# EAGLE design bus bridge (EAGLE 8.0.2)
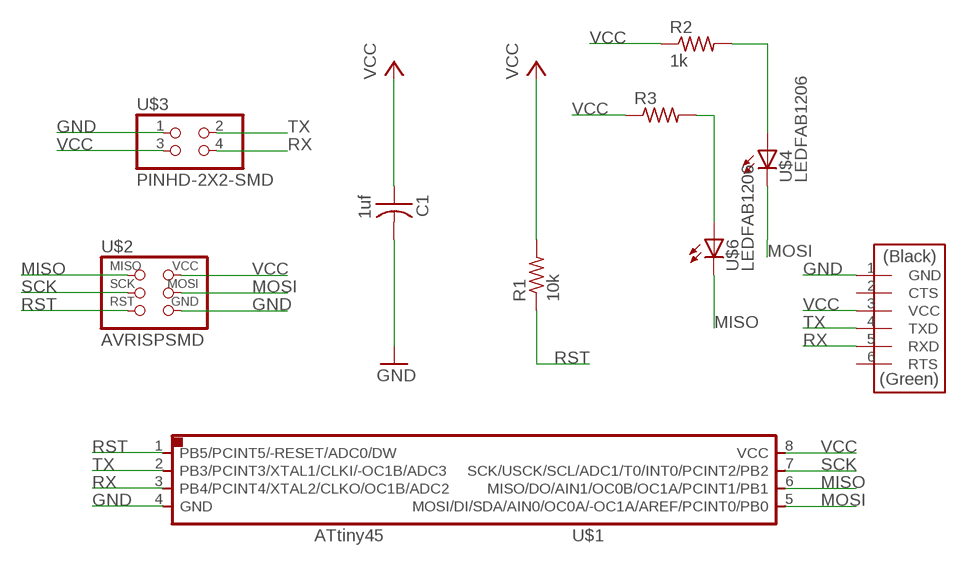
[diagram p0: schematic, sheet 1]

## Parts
C1  1uf  CAP-US1206FAB  [C1206FAB]
R1  10k  RES-US1206FAB  [R1206FAB]
R2  1k  RES-US1206FAB  [R1206FAB]
R3  RES-US1206FAB  [R1206FAB]
U$1  ATTINY45SI  [SOIC8]
U$2  AVRISPSMD  [2X03SMD]
U$3  PINHD-2X2-SMD  [2X02SMD]
U$4  LEDFAB1206  [LED1206FAB]
U$5  FTDI-SMD-HEADER  [1X06SMD]
U$6  LEDFAB1206  [LED1206FAB]

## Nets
GND: C1.2 U$1.4(GND) U$2.6(GND) U$3.1 U$5.1(GND)
MISO: U$1.6(MISO/DO/AIN1/OC0B/OC1A/PCINT1/PB1) U$2.1(MISO) U$6.2(C)
MOSI: U$1.5(MOSI/DI/SDA/AIN0/OC0A/-OC1A/AREF/PCINT0/PB0) U$2.4(MOSI) U$4.2(C)
N$2: R2.2 U$4.1(A)
N$3: R3.2 U$6.1(A)
RST: R1.1 U$1.1(PB5/PCINT5/-RESET/ADC0/DW) U$2.5(RST)
RX: U$1.3(PB4/PCINT4/XTAL2/CLKO/OC1B/ADC2) U$3.4 U$5.5(RXD)
SCK: U$1.7(SCK/USCK/SCL/ADC1/T0/INT0/PCINT2/PB2) U$2.3(SCK)
TX: U$1.2(PB3/PCINT3/XTAL1/CLKI/-OC1B/ADC3) U$3.2 U$5.4(TXD)
VCC: C1.1 R1.2 R2.1 R3.1 U$1.8(VCC) U$2.2(VCC) U$3.3 U$5.3(VCC)
Unconnected: U$5.2(CTS) U$5.6(RTS)

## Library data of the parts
C1 = fab:CAP-US
R1-R3 = fab:RES-US: Resistor (US Symbol)
U$1 = fab:ATTINY45
U$2 = fab:AVRISP
U$3 = fab:PINHD-2X2-SMD
U$4 U$6 = fab:LED: LED
U$5 = fab:FTDI-SMD-HEADER

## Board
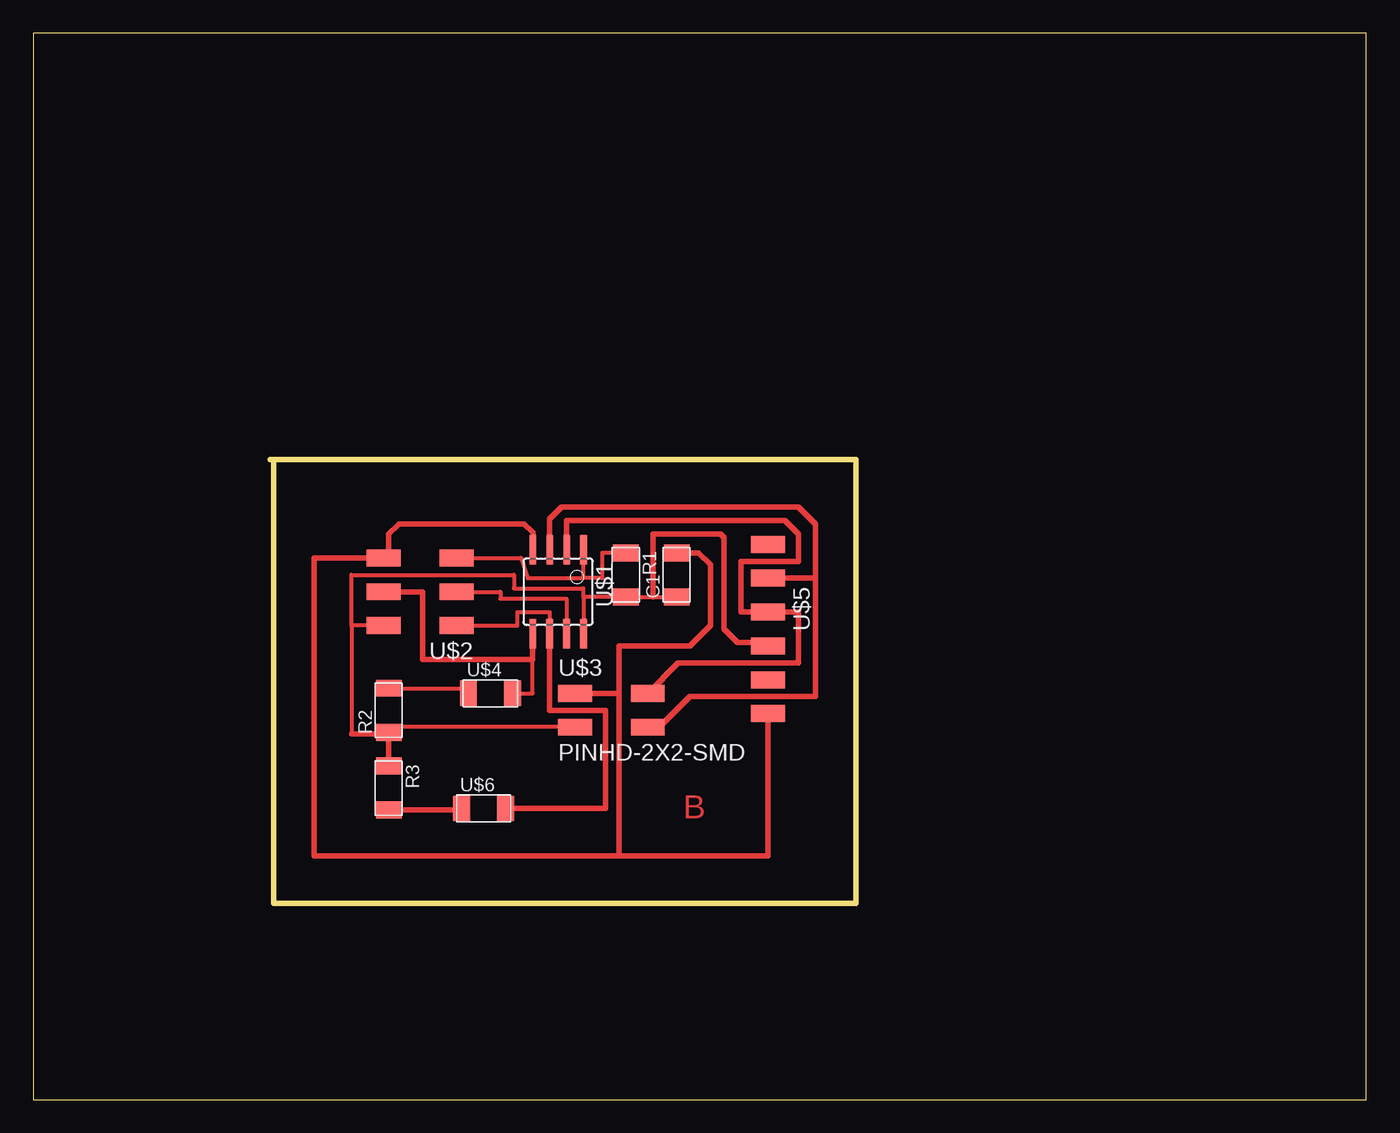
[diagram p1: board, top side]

Size 100 x 80 mm. Coordinates in mm from the lower left corner, seen from the top.
Outline: 17.78,48.01 61.72,48.01 61.72,14.73 18.03,14.73 18.03,47.75
Outline: 0,0 100,0 100,80 0,80 0,0
Copper layers (1*16): Top 0.035mm / dielectric 1.5mm / Bottom 0.035mm
Design rules "default": minimum track width 10mil, minimum drill 24mil, track to track 8mil, track to pad 8mil, pad to pad 8mil, via to via 8mil, smd to smd 8mil, copper to edge 40mil, drill to drill 8mil, minimum pad ring 10mil, minimum via ring 8mil, stop-mask expansion 4mil, vias tented up to drill 0mil, thermal gap 10mil

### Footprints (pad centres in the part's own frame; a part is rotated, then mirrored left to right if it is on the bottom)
C1206FAB = smd 1.27 x 1.905: 1 -1.651,0; 2 1.651,0
R1206FAB = smd 1.27 x 1.905: 1 -1.651,0; 2 1.651,0
SOIC8 = smd 0.5 x 2.2: 1 -1.905,-3.154; 2 -0.645,-3.154; 3 0.625,-3.154; 4 1.895,-3.154; 5 1.905,3.154; 6 0.635,3.154; 7 -0.635,3.154; 8 -1.905,3.154
2X03SMD = smd 2.54 x 1.27: 1 -2.54,2.54; 2 2.92,2.54; 3 -2.54,0; 4 2.92,0; 5 -2.54,-2.54; 6 2.92,-2.54
2X02SMD = smd 2.54 x 1.27: 1 -2.54,1.27; 2 2.92,1.27; 3 -2.54,-1.27; 4 2.92,-1.27
LED1206FAB = smd 1.27 x 1.905: 1 -1.651,0; 2 1.651,0
1X06SMD = smd 2.54 x 1.27: 1 0,6.35; 2 0,3.81; 3 0,1.27; 4 0,-1.27; 5 0,-3.81; 6 0,-6.35

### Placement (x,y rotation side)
C1  48.26,39.37 90 top
R1  44.45,39.37 270 top
R2  26.67,29.21 90 top
R3  26.67,23.37 270 top
U$1  39.37,38.1 180 top
U$2  29.21,38.1 180 top
U$3  43.18,29.21 0 top
U$4  34.29,30.48 0 top
U$5  55.12,35.31 180 top
U$6  33.78,21.84 0 top

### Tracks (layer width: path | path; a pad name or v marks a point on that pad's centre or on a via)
GND
  Top 0.406: 43.94,30.48 U$3.1 | C1.2 49.91,41.02 50.8,40.13 50.8,35.56 49.28,34.04 43.94,34.04 43.94,30.48 | U$1.4 37.48,42.53 36.83,43.18 27.43,43.18 26.67,42.42 26.67,40.64 U$2.6 21.08,40.64 21.08,18.29 43.94,18.29 | 43.94,30.48 43.94,18.29 | U$5.1 55.12,18.29 43.94,18.29
MISO
  Top 0.305: U$2.1 36.32,35.56 36.32,36.58 38.73,36.58 U$1.6
  Top 0.406: U$6.2 42.93,21.84 42.93,29.21 38.73,29.21 U$1.6
MOSI
  Top 0.305: U$4.2 37.47,30.48 37.47,33.02
  Top 0.406: U$2.4 29.21,38.1 29.21,33.02 37.47,33.02 U$1.5
N$2
  Top 0.305: R2.2 32.64,30.86 U$4.1
N$3
  Top 0.406: R3.2 32.13,21.72 U$6.1
RST
  Top 0.305: U$2.5 36.58,40.64 37.08,39.12 41.27,39.12 | 41.27,39.12 U$1.1 | R1.1 42.67,41.02 42.67,39.12 41.27,39.12
RX
  Top 0.406: U$1.3 38.74,43.57 39.62,44.45 57.4,44.45 58.67,43.18 58.67,39.12 | 58.67,39.12 58.67,30.23 49.28,30.23 46.99,27.94 U$3.4 | 58.67,39.12 U$5.5
SCK
  Top 0.305: U$2.3 35.05,38.1 35.05,37.59 40.01,37.59 U$1.7
TX
  Top 0.406: U$3.2 48.39,32.77 57.4,32.77 57.4,36.58 U$5.4 53.09,36.58 53.09,40.39 57.4,40.39 57.4,42.42 56.39,43.43 40.02,43.43 U$1.2
VCC
  Top 0.305: 23.88,35.56 23.88,39.37 36.07,39.37 36.07,38.35 41.27,38.35 41.27,37.72 | 41.27,37.72 U$1.8 | 41.27,37.72 R1.2 46.48,37.72 C1.1 | U$2.2 23.88,35.56 | 23.88,35.56 23.88,27.43 | 26.67,27.43 R2.1 26.67,27.94 U$3.3
  Top 0.406: U$5.3 54.86,34.29 52.83,34.29 51.82,35.31 51.82,42.16 51.56,42.42 46.48,42.42 46.48,37.72 | 23.88,27.43 26.67,27.43 R3.1

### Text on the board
Top: B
